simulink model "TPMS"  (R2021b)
settings: Solver=VariableStepAuto  StartTime=0.0  StopTime=10.0  RelTol=1e-3

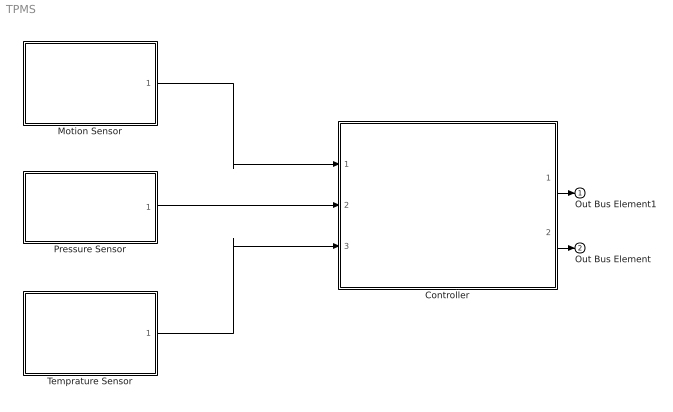
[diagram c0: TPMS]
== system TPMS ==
  Controller : Subsystem
  Motion Sensor : Subsystem
  Pressure Sensor : Subsystem
  Temprature Sensor : Subsystem
  Out Bus Element1 : Outport
  Out Bus Element : Outport  Port=2
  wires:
  Controller/2(Bus Element Out2) -> Out Bus Element/1
  Controller/1(Bus Element Out1) -> Out Bus Element1/1
  Motion Sensor/1(Bus Element Out1) -> Controller/1(Bus Element In1)
  Pressure Sensor/1(Bus Element Out1) -> Controller/2(Bus Element In2)
  Temprature Sensor/1(Bus Element Out1) -> Controller/3(Bus Element In3)

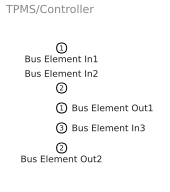
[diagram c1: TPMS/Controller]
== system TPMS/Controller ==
  Bus Element In1 : Inport
  Bus Element In2 : Inport  Port=2
  Bus Element In3 : Inport  Port=3
  Bus Element Out1 : Outport
  Bus Element Out2 : Outport  Port=2

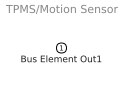
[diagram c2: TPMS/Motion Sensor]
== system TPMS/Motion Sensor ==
  Bus Element Out1 : Outport

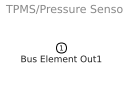
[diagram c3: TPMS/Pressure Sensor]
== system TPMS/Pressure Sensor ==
  Bus Element Out1 : Outport

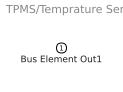
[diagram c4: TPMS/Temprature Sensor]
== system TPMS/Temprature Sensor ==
  Bus Element Out1 : Outport
